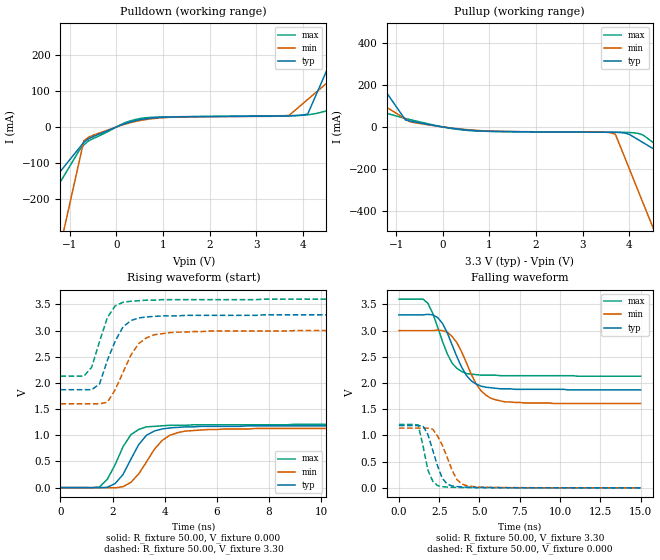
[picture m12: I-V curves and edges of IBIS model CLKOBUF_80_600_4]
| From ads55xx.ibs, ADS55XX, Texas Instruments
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|   Model CLKOBUF_80_600_4
[Model]   CLKOBUF_80_600_4
Model_type   Output
Polarity   Non-Inverting
Vmeas =   1.65V
C_comp   2pf   2pf   2pf
[Temperature Range]   50.00   0.10k   -20.00
[Voltage Range]   3.30V   3.00V   3.60V
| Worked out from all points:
|   slope of the pulldown table from 0 to 0.495 V, typ, clamps not added: 25 ohm
|   slope of the pullup table from 0 to 0.495 V, typ, clamps not added: 35.6 ohm
|   rising waveform, R_fixture 50.00, V_fixture 0.000: 20-80 % time 831ps typ, 996ps min, 757ps max; typ from 0 V to 1.18 V
|   rising waveform, R_fixture 50.00, V_fixture 3.30: 20-80 % time 720ps typ, 850ps min, 600ps max; typ from 1.87 V to 3.3 V
|   falling waveform, R_fixture 50.00, V_fixture 3.30: 20-80 % time 1.26ns typ, 1.33ns min, 1.1ns max; typ from 3.3 V to 1.87 V
|   falling waveform, R_fixture 50.00, V_fixture 0.000: 20-80 % time 759ps typ, 955ps min, 565ps max; typ from 1.19 V to 0.001 V
[Pulldown]
| voltage   I(typ)   I(min)   I(max)
-3.3V     -458.6mA   -1.545A    -606.7mA
-2.1V     -266.7mA   -849.9mA   -346.9mA
-1.7V     -202.7mA   -618.2mA   -260.3mA
-1.5V     -170.8mA   -502.4mA   -217mA
-1V       -90.8mA    -212.8mA   -108.7mA
-700mV    -42.83mA   -39mA      -49.96mA
300mV     13.85mA    11.85mA    16.87mA
3.7V      30.36mA    31.86mA    31.32mA
4.1V      35.53mA    76.1mA     33.57mA
4.9V      272.4mA    164.6mA    57.52mA
5.9V      568.5mA    275.2mA    90.47mA
6.6V      775.8mA    352.6mA    113.5mA
[Pullup]
| voltage   I(typ)   I(min)   I(max)
-3.3V     837.4mA    380.4mA    192.5mA
-2.3V     515.7mA    243.5mA    131.6mA
-2.1V     451.4mA    216.1mA    119.4mA
-800mV    33.19mA    38.16mA    40.27mA
-600mV    23.75mA    20.33mA    29.67mA
600mV     -15.96mA   -14.36mA   -17.86mA
3.6V      -25.18mA   -27.56mA   -25.55mA
3.7V      -25.4mA    -34.74mA   -25.65mA
4V        -35.63mA   -200.4mA   -26.55mA
4.2V      -62.27mA   -310.8mA   -31.5mA
4.5V      -102.2mA   -476.5mA   -72.82mA
6.6V      -382mA     -1.636A    -421.1mA
[Ramp]
| variable   typ   min   max
dV/dt_r   0.71/0.80n   0.68/0.96n   0.72/0.71n
dV/dt_f   0.86/1.24n   0.84/1.32n   0.88/1.07n
R_load = 50.00
[Rising Waveform]
R_fixture = 50.00
V_fixture = 0.000
V_fixture_min = 0.000
V_fixture_max = 0.000
| time   V(typ)   V(min)   V(max)
0s        27.81nV    35.94nV    54.86nV
1.5ns     -3.03mV    33.65uV    14.22mV
1.8ns     5.46mV     -2.15mV    160mV
2.1ns     78.14mV    -5.03mV    440mV
2.4ns     250mV      17.48mV    780mV
2.7ns     540mV      100mV      1.01V
3.3ns     1V         490mV      1.16V
3.9ns     1.12V      900mV      1.18V
4.8ns     1.16V      1.08V      1.19V
15ns      1.18V      1.14V      1.21V
[Rising Waveform]
R_fixture = 50.00
V_fixture = 3.30
V_fixture_min = 3.00
V_fixture_max = 3.60
| time   V(typ)   V(min)   V(max)
0s        1.87V      1.6V       2.13V
900ps     1.87V      1.6V       2.13V
1.2ns     1.87V      1.6V       2.3V
1.5ns     1.98V      1.6V       2.79V
1.8ns     2.43V      1.63V      3.25V
2.1ns     2.8V       1.87V      3.47V
2.4ns     3.07V      2.2V       3.54V
3ns       3.24V      2.75V      3.57V
4.2ns     3.28V      2.96V      3.59V
15ns      3.3V       3V         3.6V
[Falling Waveform]
R_fixture = 50.00
V_fixture = 3.30
V_fixture_min = 3.00
V_fixture_max = 3.60
| time   V(typ)   V(min)   V(max)
0s        3.3V       3V         3.6V
1.5ns     3.3V       3V         3.6V
1.8ns     3.31V      3V         3.52V
2.4ns     3.25V      3.01V      3.07V
2.7ns     3.14V      3V         2.8V
3.3ns     2.73V      2.89V      2.38V
4.2ns     2.14V      2.38V      2.18V
5.1ns     1.94V      1.85V      2.15V
6ns       1.9V       1.68V      2.15V
15ns      1.87V      1.61V      2.13V
[Falling Waveform]
R_fixture = 50.00
V_fixture = 0.000
V_fixture_min = 0.000
V_fixture_max = 0.000
| time   V(typ)   V(min)   V(max)
0s        1.19V      1.14V      1.21V
1.2ns     1.19V      1.14V      1.2V
1.5ns     1.18V      1.14V      800mV
1.8ns     1.02V      1.14V      340mV
2.4ns     420mV      990mV      43.93mV
2.7ns     180mV      810mV      23.97mV
3ns       73.05mV    580mV      16.55mV
3.6ns     25.55mV    160mV      9.57mV
4.2ns     13.79mV    42.99mV    6.75mV
15ns      1.12mV     1.41mV     1.13mV
